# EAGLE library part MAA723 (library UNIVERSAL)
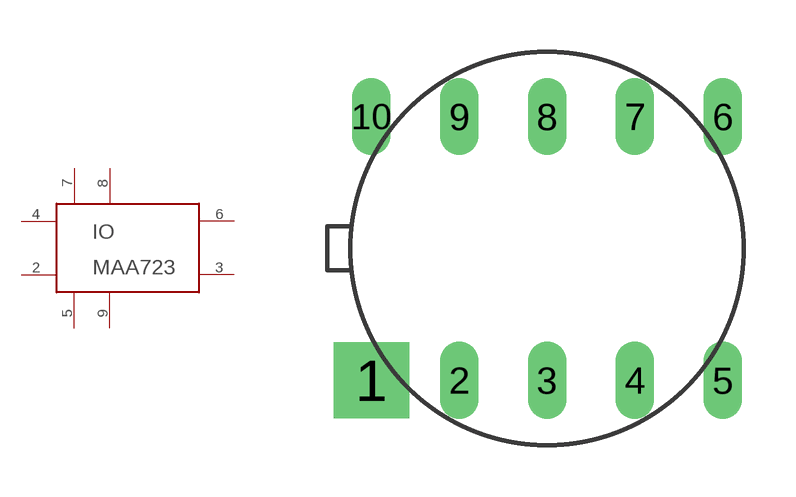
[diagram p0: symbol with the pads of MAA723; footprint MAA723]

Designator prefix IO

## MAA723  [MAA723]
2  2
3  3
4  4
5  5
6  6
7  7
8  8
9  9

## Footprint MAA723 (pad centres in mm)
drill 0.61 pad 2.184 square: 1 0,0
drill 0.61 pad 1.092 long: 2 2.54,0; 3 5.08,0; 4 7.62,0; 5 10.16,0; 6 10.16,7.62; 7 7.62,7.62; 8 5.08,7.62; 9 2.54,7.62; 10 0,7.62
